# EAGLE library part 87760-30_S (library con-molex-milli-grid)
HEADER
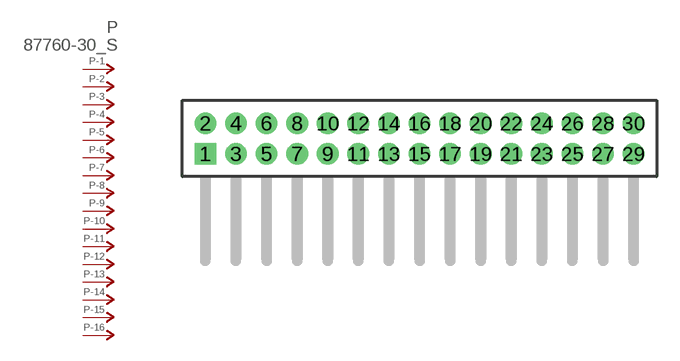
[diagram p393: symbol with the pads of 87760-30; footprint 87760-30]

Designator prefix P; gates -1=P-NV -2=P-N -3=P-N -4=P-N -5=P-N -6=P-N -7=P-N -8=P-N -9=P-N -10=P-N -11=P-N -12=P-N -13=P-N -14=P-N -15=P-N -16=P-N -17=P-N -18=P-N -19=P-N -20=P-N -21=P-N -22=P-N -23=P-N -24=P-N -25=P-N -26=P-N -27=P-N -28=P-N -29=P-N -30=P-N

## 87760-30_S  [87760-30]
1  -1:P  pas
2  -2:P  pas
3  -3:P  pas
4  -4:P  pas
5  -5:P  pas
6  -6:P  pas
7  -7:P  pas
8  -8:P  pas
9  -9:P  pas
10  -10:P  pas
11  -11:P  pas
12  -12:P  pas
13  -13:P  pas
14  -14:P  pas
15  -15:P  pas
16  -16:P  pas
17  -17:P  pas
18  -18:P  pas
19  -19:P  pas
20  -20:P  pas
21  -21:P  pas
22  -22:P  pas
23  -23:P  pas
24  -24:P  pas
25  -25:P  pas
26  -26:P  pas
27  -27:P  pas
28  -28:P  pas
29  -29:P  pas
30  -30:P  pas

## Footprint 87760-30 (pad centres in mm)
HEADER Dual Row, Right Angle
drill 0.914 square: 1 -14,-1
drill 0.914: 2 -14,1; 3 -12,-1; 4 -12,1; 5 -10,-1; 6 -10,1; 7 -8,-1; 8 -8,1; 9 -6,-1; 10 -6,1; 11 -4,-1; 12 -4,1; 13 -2,-1; 14 -2,1; 15 0,-1; 16 0,1; 17 2,-1; 18 2,1; 19 4,-1; 20 4,1; 21 6,-1; 22 6,1; 23 8,-1; 24 8,1; 25 10,-1; 26 10,1; 27 12,-1; 28 12,1; 29 14,-1; 30 14,1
